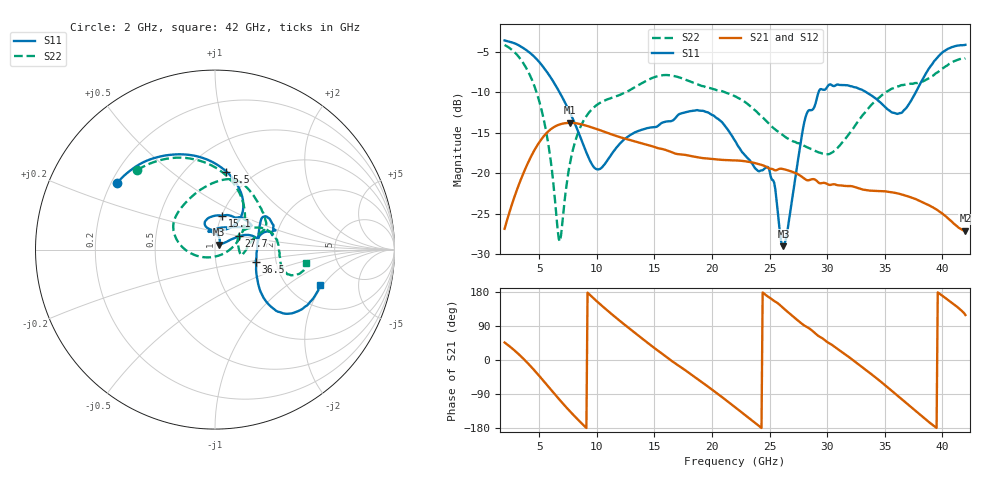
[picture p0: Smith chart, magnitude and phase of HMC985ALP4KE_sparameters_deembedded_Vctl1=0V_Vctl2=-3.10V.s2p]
!s2p File: Measurements: S11, S21, S12, S22
# GHz S dB R 50.0
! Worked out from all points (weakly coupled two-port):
!   401 points, 2 GHz to 42 GHz, reference 50 ohm
!   highest |S21| = -13.77 dB at 7.7 GHz (marker M1); lowest = -27.1 dB at 42 GHz (marker M2)
!   lowest |S11| = -29.0 dB at 26.2 GHz (marker M3), VSWR 1.07, Z = 52.3 + j2.84 ohm
!   |S11| at or under -10 dB: 6.768 GHz to 29.25 GHz (22.49 GHz wide, 125 % of centre); 33.4 GHz to 37.7 GHz (4.295 GHz wide, 12.1 % of centre)
!   |S22| runs from -28.4 to -4.2 dB; largest |S21 - S12| = 0.00063
!   S11 on the Smith chart (normalised r, x): 2 GHz: 0.22, +0.29; 5.5 GHz: 0.76, +0.82; 15.1 GHz: 1.00, +0.39; 27.7 GHz: 1.29, +0.20; 36.5 GHz: 1.57, -0.22; 42 GHz: 2.93, -1.90
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2  -3.61 145.7  -26.86 46.2  -26.84 46.2  -4.16 134.2
3.6  -4.52 118.1  -20.10 4.3  -20.11 4.3  -6.37 94.8
5.5  -7.16 81.6  -15.26 -59.5  -15.27 -59.5  -14.06 36.7
6.7  -9.83 61.4  -14.01 -102.5  -14.01 -102.5  -28.09 -58.3
7.7  -12.59 51.8  -13.77 -136.3  -13.78 -136.3  -18.58 -165.2
8.7  -16.00 53.5  -13.97 -167.6  -13.97 -167.6  -13.92 170.6
10.2  -19.50 89.5  -14.64 149.7  -14.62 149.7  -11.38 149.4
12.4  -15.79 110.6  -15.71 93.6  -15.69 93.6  -10.07 118.8
15.1  -14.29 78.2  -16.79 29.3  -16.81 29.3  -8.08 82.4
15.4  -14.06 74.6  -16.93 22.7  -16.96 22.6  -7.97 79.4
19.2  -12.29 33.6  -18.13 -60.1  -18.13 -60.1  -9.25 42.3
22  -15.98 52.0  -18.41 -124.4  -18.42 -124.4  -10.49 22.3
25  -19.71 99.7  -19.43 164.5  -19.43 164.4  -13.96 10.9
26.2  -29.00 49.9  -19.49 136.8  -19.49 136.8  -15.36 -1.6
27.7  -16.27 28.9  -20.32 98.2  -20.36 98.2  -16.42 -11.8
28.7  -12.18 12.9  -20.73 77.4  -20.70 77.4  -17.04 -8.1
31  -9.06 23.2  -21.49 27.0  -21.48 27.0  -16.71 28.0
33.3  -9.91 34.2  -22.06 -24.9  -22.07 -24.9  -12.47 30.7
35.4  -12.25 11.8  -22.30 -76.0  -22.31 -76.1  -9.75 17.1
36.5  -12.50 -16.5  -22.63 -104.5  -22.61 -104.5  -9.11 8.4
39.5  -5.84 -43.5  -24.48 -179.3  -24.50 -179.3  -7.60 -18.0
42  -4.15 -18.8  -27.08 118.8  -27.12 118.8  -5.81 -8.6
